[IBIS Ver]   3.2
[File name]   apollo7a.ibs
[File Rev]   0.2
[Date]   Wed Oct 23 16:15:15 CDT 2002
[Source]   File originated at Motorola Somerset Design Center.
|   Created by Jim Nissen.
[Notes]   This IBIS model is for the Apollo7 360CBGA ceramic package.
|   The driver and receiver models are characterized up to
|   2.5V mode on the data bus and 2.5V mode on the L3
|   interface. The convention is apollox.ibs, where x
|   is one of the configurations of data bus/L3 bus voltage
|   modes. Following is a table of the code for bus combinations:
|   IBIS model   Bus mode   L3 mode
|   apollo7a.ibs   2.5V   2.5V
|   apollo7b.ibs   2.5V   1.8V
|   apollo7c.ibs   2.5V   1.5V
|   apollo7d.ibs   1.8V   2.5V
|   apollo7e.ibs   1.8V   1.8V
|   apollo7f.ibs   1.8V   1.5V
|   apollo7g.ibs   1.5V   2.5V
|   apollo7h.ibs   1.5V   1.8V
|   apollo7i.ibs   1.5V   1.5V
[Disclaimer]   This information is for modeling purposes only and
|   is not guaranteed.
[Component]   Apollo7
[Manufacturer]  Motorola
[Package]
|   typ   min   max
R_pkg   0.0   0.0   0.0
L_pkg   0.0   0.0   0.0
C_pkg   0.0   0.0   0.0
[Pin]   signal_name   model_name   R_pin   L_pin   C_pin
A2   SRESET_B   busio   1E-016   1E-016   1E-016
A3   CKSTP_IN_B   busio   1E-016   1E-016   1E-016
A4   TDO   busio   1E-016   1E-016   1E-016
A5   TRST_B   rcvr   1E-016   1E-016   1E-016
A6   HPR_B   busio   1E-016   1E-016   1E-016
A7   PLL_CFG(4)   busio   1E-016   1E-016   1E-016
A9   PMON_OUT_B   busio   1E-016   1E-016   1E-016
A10   SYSCLK   busio   1E-016   1E-016   1E-016
A11   EXT_QUAL   busio   1E-016   1E-016   1E-016
A12   CHKS_B   busio   1E-016   1E-016   1E-016
A13   L3_DATA(59)   l3io   1E-016   1E-016   1E-016
A14   L3_DATA(61)   l3io   1E-016   1E-016   1E-016
A15   L3_DATA(56)   l3io   1E-016   1E-016   1E-016
A16   L3_DATA(36)   l3io   1E-016   1E-016   1E-016
A17   L3_DATA(50)   l3io   1E-016   1E-016   1E-016
A18   L3_DATA(58)   l3io   1E-016   1E-016   1E-016
A19   L3_DATA(38)   l3io   1E-016   1E-016   1E-016
B1   CKSTP_OUT_B   busio   1E-016   1E-016   1E-016
B2   HIT_B   busio   1E-016   1E-016   1E-016
B3   L2_TSTCLK   rcvr   1E-016   1E-016   1E-016
B6   IARTRY0_B   busio   1E-016   1E-016   1E-016
B7   BVSEL   rcvr   1E-016   1E-016   1E-016
B8   PLL_CFG(0)   busio   1E-016   1E-016   1E-016
B9   TDI   rcvr   1E-016   1E-016   1E-016
B10   SRW_B(0)   busio   1E-016   1E-016   1E-016
B11   A(35)   busio   1E-016   1E-016   1E-016
B12   A(32)   busio   1E-016   1E-016   1E-016
B13   L3_DATAP(6)   l3io   1E-016   1E-016   1E-016
B14   L3_DATAP(7)   l3io   1E-016   1E-016   1E-016
B15   L3_DATA(41)   l3io   1E-016   1E-016   1E-016
B16   L3_DATA(55)   l3io   1E-016   1E-016   1E-016
B17   L3_DATA(42)   l3io   1E-016   1E-016   1E-016
B18   L3_DATAP(4)   l3io   1E-016   1E-016   1E-016
B19   L3_DATA(37)   l3io   1E-016   1E-016   1E-016
C1   AP(0)   busio   1E-016   1E-016   1E-016
C4   A(33)   busio   1E-016   1E-016   1E-016
C5   TT(4)   busio   1E-016   1E-016   1E-016
C6   TCK   rcvr   1E-016   1E-016   1E-016
C7   PLL_CFG(2)   busio   1E-016   1E-016   1E-016
C8   PLL_CFG(1)   busio   1E-016   1E-016   1E-016
C9   MCP_B   busio   1E-016   1E-016   1E-016
C10   A(8)   busio   1E-016   1E-016   1E-016
C11   A(2)   busio   1E-016   1E-016   1E-016
C13   L3_DATA(63)   l3io   1E-016   1E-016   1E-016
C14   L3_DATA(57)   l3io   1E-016   1E-016   1E-016
C15   L3_DATA(49)   l3io   1E-016   1E-016   1E-016
C16   L3_DATA(44)   l3io   1E-016   1E-016   1E-016
C17   L3_DATA(43)   l3io   1E-016   1E-016   1E-016
C18   L3_DATA(35)   l3io   1E-016   1E-016   1E-016
C19   L3_DATA(32)   l3io   1E-016   1E-016   1E-016
D1   A(7)   busio   1E-016   1E-016   1E-016
D2   BR_B   busio   1E-016   1E-016   1E-016
D3   WT_B   busio   1E-016   1E-016   1E-016
D4   INT_B   busio   1E-016   1E-016   1E-016
D7   PLL_CFG(3)   busio   1E-016   1E-016   1E-016
D8   HRESET_B   busio   1E-016   1E-016   1E-016
D9   PMON_IN_B   busio   1E-016   1E-016   1E-016
D10   DX_B   busio   1E-016   1E-016   1E-016
D11   A(6)   busio   1E-016   1E-016   1E-016
D12   A(10)   busio   1E-016   1E-016   1E-016
D14   L3_DATA(39)   l3io   1E-016   1E-016   1E-016
D15   L3_DATA(33)   l3io   1E-016   1E-016   1E-016
D16   L3_ADDR(16)   l3io   1E-016   1E-016   1E-016
D17   L3_ADDR(15)   l3io   1E-016   1E-016   1E-016
D18   L3_ADDR(8)"   l3io   1E-016   1E-016   1E-016
D19   L3_ADDR(11)   l3io   1E-016   1E-016   1E-016
E1   TBEN   busio   1E-016   1E-016   1E-016
E2   GBL_B   busio   1E-016   1E-016   1E-016
E3   AP(1)   busio   1E-016   1E-016   1E-016
E4   SHD0_B   busio   1E-016   1E-016   1E-016
E5   TT(0)   busio   1E-016   1E-016   1E-016
E6   TT(1)   busio   1E-016   1E-016   1E-016
E7   TSIZ(2)   busio   1E-016   1E-016   1E-016
E8   LSSD_MODE_B   rcvr   1E-016   1E-016   1E-016
E9   TT(3)   busio   1E-016   1E-016   1E-016
E10   SRW_B(1)   busio   1E-016   1E-016   1E-016
E11   A(0)   busio   1E-016   1E-016   1E-016
E12   L3_DATAP(5)   l3io   1E-016   1E-016   1E-016
E13   L3_DATA(54)   l3io   1E-016   1E-016   1E-016
E14   L3_DATA(46)   l3io   1E-016   1E-016   1E-016
E15   L3_DATA(40)   l3io   1E-016   1E-016   1E-016
E16   L3_ADDR(14)   l3io   1E-016   1E-016   1E-016
E19   L3_ADDR(7)   l3io   1E-016   1E-016   1E-016
F1   TMS   rcvr   1E-016   1E-016   1E-016
F4   A(14)   busio   1E-016   1E-016   1E-016
F5   AP(3)   busio   1E-016   1E-016   1E-016
F6   TT(2)   busio   1E-016   1E-016   1E-016
F7   TSIZ(1)   busio   1E-016   1E-016   1E-016
F8   BMODE_B(1)   busio   1E-016   1E-016   1E-016
F9   SMI_B   busio   1E-016   1E-016   1E-016
F10   A(4)   busio   1E-016   1E-016   1E-016
F11   TBST_B   busio   1E-016   1E-016   1E-016
F12   L3_DATA(60)   l3io   1E-016   1E-016   1E-016
F13   L3_DATA(53)   l3io   1E-016   1E-016   1E-016
F14   L3_DATA(52)   l3io   1E-016   1E-016   1E-016
F15   L3_ADDR(12)   l3io   1E-016   1E-016   1E-016
F16   L3_ADDR(9)   l3io   1E-016   1E-016   1E-016
F17   L3_ADDR(1)   l3io   1E-016   1E-016   1E-016
F18   L3_ADDR(0)   l3io   1E-016   1E-016   1E-016
F19   L3_ADDR(2)   l3io   1E-016   1E-016   1E-016
G1   DTI(0)   busio   1E-016   1E-016   1E-016
G2   A(9)   busio   1E-016   1E-016   1E-016
G3   A(3)   busio   1E-016   1E-016   1E-016
G4   A(12)   busio   1E-016   1E-016   1E-016
G5   QACK_B   busio   1E-016   1E-016   1E-016
G6   TSIZ(0)   busio   1E-016   1E-016   1E-016
G7   AP(4)   busio   1E-016   1E-016   1E-016
G8   L1_TSTCLK   rcvr   1E-016   1E-016   1E-016
G9   BMODE_B(0)   busio   1E-016   1E-016   1E-016
G10   A(34)   busio   1E-016   1E-016   1E-016
G11   L3_DATA(62)   l3io   1E-016   1E-016   1E-016
G12   L3_DATA(51)   l3io   1E-016   1E-016   1E-016
G13   L3_DATA(45)   l3io   1E-016   1E-016   1E-016
G14   L3_DATA(48)   l3io   1E-016   1E-016   1E-016
G15   L3_DATA(34)   l3io   1E-016   1E-016   1E-016
G16   L3_ADDR(10)   l3io   1E-016   1E-016   1E-016
G19   L3_ADDR(13)   l3io   1E-016   1E-016   1E-016
H1   A(1)   busio   1E-016   1E-016   1E-016
H2   CLK_OUT   busio   1E-016   1E-016   1E-016
H5   SHD1_B   busio   1E-016   1E-016   1E-016
H6   AP(2)   busio   1E-016   1E-016   1E-016
H14   L3_DATA(47)   l3io   1E-016   1E-016   1E-016
H15   L3_DATA(23)   l3io   1E-016   1E-016   1E-016
H16   L3_ADDR(6)   l3io   1E-016   1E-016   1E-016
H17   L3_ADDR(5)   l3io   1E-016   1E-016   1E-016
H18   L3_ADDR(4)   l3io   1E-016   1E-016   1E-016
H19   L3_ADDR(3)   l3io   1E-016   1E-016   1E-016
J1   CI_B   busio   1E-016   1E-016   1E-016
J2   A(20)   busio   1E-016   1E-016   1E-016
J3   A(23)   busio   1E-016   1E-016   1E-016
J4   A(16)   busio   1E-016   1E-016   1E-016
J14   L3_DATA(17)   l3io   1E-016   1E-016   1E-016
J15   L3_DATA(20)   l3io   1E-016   1E-016   1E-016
J16   L3_DATA(22)   l3io   1E-016   1E-016   1E-016
J17   L3_DATA(30)   l3io   1E-016   1E-016   1E-016
J18   L3_DATA(18)   l3io   1E-016   1E-016   1E-016
J19   L3_DATA(19)   l3io   1E-016   1E-016   1E-016
K1   DTI(1)   busio   1E-016   1E-016   1E-016
K4   A(21)   busio   1E-016   1E-016   1E-016
K5   A(18)   busio   1E-016   1E-016   1E-016
K6   TA_B   busio   1E-016   1E-016   1E-016
K15   L3_DATA(16)   l3io   1E-016   1E-016   1E-016
K16   L3_DATA(31)   l3io   1E-016   1E-016   1E-016
K17   L3_DATAP(2)   l3io   1E-016   1E-016   1E-016
K18   L3_DATA(29)   l3io   1E-016   1E-016   1E-016
K19   L3_DATA(21)   l3io   1E-016   1E-016   1E-016
L1   TEA_B   busio   1E-016   1E-016   1E-016
L2   A(5)   busio   1E-016   1E-016   1E-016
L3   A(11)   busio   1E-016   1E-016   1E-016
L4   TS_B   busio   1E-016   1E-016   1E-016
L14   L3_DATA(15)   l3io   1E-016   1E-016   1E-016
L15   L3_DATA(1)   l3io   1E-016   1E-016   1E-016
L16   L3_DATA(24)   l3io   1E-016   1E-016   1E-016
L17   L3_DATA(14)   l3io   1E-016   1E-016   1E-016
L18   L3_DATA(28)   l3io   1E-016   1E-016   1E-016
L19   L3_DATA(27)   l3io   1E-016   1E-016   1E-016
M1   BG_B   busio   1E-016   1E-016   1E-016
M2   DBG_B   busio   1E-016   1E-016   1E-016
M5   A(24)   busio   1E-016   1E-016   1E-016
M6   DP(4)   busio   1E-016   1E-016   1E-016
M14   L3_DATA(5)   l3io   1E-016   1E-016   1E-016
M15   L3_DATA(13)   l3io   1E-016   1E-016   1E-016
M16   L3_DATA(10)   l3io   1E-016   1E-016   1E-016
M17   L3_DATA(6)   l3io   1E-016   1E-016   1E-016
M18   L3_DATA(26)   l3io   1E-016   1E-016   1E-016
M19   L3_DATA(9)   l3io   1E-016   1E-016   1E-016
N1   DTI(3)   busio   1E-016   1E-016   1E-016
N2   ARTRY_B   busio   1E-016   1E-016   1E-016
N3   A(26)   busio   1E-016   1E-016   1E-016
N4   A(22)   busio   1E-016   1E-016   1E-016
N5   A(30)   busio   1E-016   1E-016   1E-016
N8   DP(6)   busio   1E-016   1E-016   1E-016
N9   D(25)   busio   1E-016   1E-016   1E-016
N10   D(19)   busio   1E-016   1E-016   1E-016
N11   D(18)   busio   1E-016   1E-016   1E-016
N12   L3_DATAP(0)   l3io   1E-016   1E-016   1E-016
N13   L3_DATA(7)   l3io   1E-016   1E-016   1E-016
N14   L3_DATA(4)   l3io   1E-016   1E-016   1E-016
N15   L3_DATA(2)   l3io   1E-016   1E-016   1E-016
N16   L3_DATA(8)   l3io   1E-016   1E-016   1E-016
N17   L3_DATA(12)   l3io   1E-016   1E-016   1E-016
N18   L3_DATAP(1)   l3io   1E-016   1E-016   1E-016
N19   L3_DATAP(3)   l3io   1E-016   1E-016   1E-016
P1   DTI(2)   busio   1E-016   1E-016   1E-016
P4   QREQ_B   busio   1E-016   1E-016   1E-016
P5   A(25)   busio   1E-016   1E-016   1E-016
P6   D(60)   busio   1E-016   1E-016   1E-016
P7   D(38)   busio   1E-016   1E-016   1E-016
P10   D(26)   busio   1E-016   1E-016   1E-016
P13   D(11)   busio   1E-016   1E-016   1E-016
P14   D(7)   busio   1E-016   1E-016   1E-016
P15   L3_DATA(0)   l3io   1E-016   1E-016   1E-016
P16   L3_DATA(25)   l3io   1E-016   1E-016   1E-016
P17   D(40)   busio   1E-016   1E-016   1E-016
P18   L3_DATA(3)   l3io   1E-016   1E-016   1E-016
P19   L3_DATA(11)   l3io   1E-016   1E-016   1E-016
R1   AACK_B   busio   1E-016   1E-016   1E-016
R2   A(17)   busio   1E-016   1E-016   1E-016
R3   DRDY_B   busio   1E-016   1E-016   1E-016
R6   D(37)   busio   1E-016   1E-016   1E-016
R7   D(59)   busio   1E-016   1E-016   1E-016
R8   D(61)   busio   1E-016   1E-016   1E-016
R9   D(28)   busio   1E-016   1E-016   1E-016
R10   D(24)   busio   1E-016   1E-016   1E-016
R11   D(20)   busio   1E-016   1E-016   1E-016
R12   D(14)   busio   1E-016   1E-016   1E-016
R15   D(0)   busio   1E-016   1E-016   1E-016
R18   D(43)   busio   1E-016   1E-016   1E-016
R19   D(41)   busio   1E-016   1E-016   1E-016
T1   A(27)   busio   1E-016   1E-016   1E-016
T2   A(13)   busio   1E-016   1E-016   1E-016
T3   DP(0)   busio   1E-016   1E-016   1E-016
T4   DP(2)   busio   1E-016   1E-016   1E-016
T5   D(34)   busio   1E-016   1E-016   1E-016
T8   D(63)   busio   1E-016   1E-016   1E-016
T11   D(23)   busio   1E-016   1E-016   1E-016
T12   D(15)   busio   1E-016   1E-016   1E-016
T13   D(10)   busio   1E-016   1E-016   1E-016
T14   D(2)   busio   1E-016   1E-016   1E-016
T15   D(5)   busio   1E-016   1E-016   1E-016
T16   D(51)   busio   1E-016   1E-016   1E-016
T17   D(53)   busio   1E-016   1E-016   1E-016
T18   D(52)   busio   1E-016   1E-016   1E-016
T19   D(45)   busio   1E-016   1E-016   1E-016
U1   A(29)   busio   1E-016   1E-016   1E-016
U4   D(56)   busio   1E-016   1E-016   1E-016
U5   D(35)   busio   1E-016   1E-016   1E-016
U6   D(33)   busio   1E-016   1E-016   1E-016
U7   D(58)   busio   1E-016   1E-016   1E-016
U8   D(57)   busio   1E-016   1E-016   1E-016
U9   D(30)   busio   1E-016   1E-016   1E-016
U10   D(27)   busio   1E-016   1E-016   1E-016
U11   D(21)   busio   1E-016   1E-016   1E-016
U14   D(12)   busio   1E-016   1E-016   1E-016
U15   D(6)   busio   1E-016   1E-016   1E-016
U18   D(48)   busio   1E-016   1E-016   1E-016
U19   D(46)   busio   1E-016   1E-016   1E-016
V1   A(15)   busio   1E-016   1E-016   1E-016
V2   A(28)   busio   1E-016   1E-016   1E-016
V3   DP(5)   busio   1E-016   1E-016   1E-016
V6   D(39)   busio   1E-016   1E-016   1E-016
V9   D(31)   busio   1E-016   1E-016   1E-016
V12   D(17)   busio   1E-016   1E-016   1E-016
V13   D(8)   busio   1E-016   1E-016   1E-016
V16   D(3)   busio   1E-016   1E-016   1E-016
V17   D(55)   busio   1E-016   1E-016   1E-016
V18   D(42)   busio   1E-016   1E-016   1E-016
V19   D(44)   busio   1E-016   1E-016   1E-016
W1   A(31)   busio   1E-016   1E-016   1E-016
W2   A(19)   busio   1E-016   1E-016   1E-016
W3   D(54)   busio   1E-016   1E-016   1E-016
W4   DP(1)   busio   1E-016   1E-016   1E-016
W5   D(32)   busio   1E-016   1E-016   1E-016
W6   DP(7)   busio   1E-016   1E-016   1E-016
W7   D(36)   busio   1E-016   1E-016   1E-016
W8   D(62)   busio   1E-016   1E-016   1E-016
W9   DP(3)   busio   1E-016   1E-016   1E-016
W10   D(29)   busio   1E-016   1E-016   1E-016
W11   D(22)   busio   1E-016   1E-016   1E-016
W12   D(16)   busio   1E-016   1E-016   1E-016
W13   D(9)   busio   1E-016   1E-016   1E-016
W14   D(13)   busio   1E-016   1E-016   1E-016
W15   D(1)   busio   1E-016   1E-016   1E-016
W16   D(4)   busio   1E-016   1E-016   1E-016
W17   D(49)   busio   1E-016   1E-016   1E-016
W18   D(50)   busio   1E-016   1E-016   1E-016
W19   D(47)   busio   1E-016   1E-016   1E-016
|!!!![Package Model] 'name'  calls name
[Package Model] apollo7_360
[Define Package Model] apollo7_360
[Manufacturer] Motorola Inc.
[OEM] Motorola Inc.
[Description] Apollo7 360 CBGA Package T-Line pkg model
[Number Of Sections] 10
[Number Of Pins]  267
[Pin Numbers]
|Although any length unit can be used for Len, mm is used here.
|signal (1)SYSCLK
A10   Len=0 L=0.023752784n /
Len=0 L=0.0115888305n /
Len=10.910172 L=0.41228828n C=0.27619976p R=0.045776114 /
Len=0 L=0.0115888305n /
Len=0 L=0.0115888305n /
Len=0 L=0.0115888305n /
Len=0 L=0.0115888305n /
Len=0 L=0.027n /
|signal (2)EXT_QUAL
A11   Len=0 L=0.023752784n /
Len=0 L=0.0115888305n /
Len=10.207413 L=0.41011378n C=0.27773488p R=0.04516712 /
Len=0 L=0.0115888305n /
Len=0 L=0.0115888305n /
Len=0 L=0.0115888305n /
Len=0 L=0.0115888305n /
Len=0 L=0.027n /
|signal (3)CHKS_B
A12   Len=0 L=0.023752784n /
Len=0 L=0.0115888305n /
Len=0 L=0.0115888305n /
Len=0 L=0.0115888305n /
Len=12.901163 L=0.4005851n C=0.2846683p R=0.04260898 /
Len=0 L=0.0115888305n /
Len=0 L=0.0115888305n /
Len=0 L=0.027n /
|signal (4)L3_DATA(59)
A13   Len=0 L=0.023752784n /
Len=0 L=0.0115888305n /
Len=0 L=0.0115888305n /
Len=0 L=0.0115888305n /
Len=5.8014994 L=0.42097718n C=0.2702314p R=0.04830918 /
Len=0 L=0.0115888305n /
Len=0 L=0.0115888305n /
Len=5.8287997 L=0.4658248n C=0.12673753p R=0.041152265 /
Len=0 L=0.027n /
|signal (5)L3_DATA(61)
A14   Len=0 L=0.023752784n /
Len=0 L=0.0115888305n /
Len=11.64697 L=0.40967372n C=0.27804765p R=0.045045044 /
Len=0 L=0.0115888305n /
Len=0 L=0.0115888305n /
Len=0 L=0.0115888305n /
Len=0 L=0.0115888305n /
Len=0 L=0.027n /
|signal (6)L3_DATA(56)
A15   Len=0 L=0.023752784n /
Len=0 L=0.0115888305n /
Len=0 L=0.0115888305n /
Len=0 L=0.0115888305n /
Len=0 L=0.0115888305n /
Len=0 L=0.0115888305n /
Len=14.642346 L=0.4886838n C=0.120809175p R=0.047340576 /
Len=0 L=0.027n /
|signal (7)L3_DATA(36)
A16   Len=0 L=0.023752784n /
Len=0 L=0.0115888305n /
Len=0 L=0.0115888305n /
Len=0 L=0.0115888305n /
Len=9.291906 L=0.41293234n C=0.27574828p R=0.045958366 /
Len=0 L=0.0115888305n /
Len=0 L=0.0115888305n /
Len=5.9719596 L=0.4658248n C=0.12673753p R=0.041152265 /
Len=0 L=0.027n /
|signal (8)L3_DATA(50)
A17   Len=0 L=0.023752784n /
Len=0 L=0.0115888305n /
Len=0 L=0.0115888305n /
Len=0 L=0.0115888305n /
Len=0 L=0.0115888305n /
Len=0 L=0.0115888305n /
Len=17.10347 L=0.4950636n C=0.119252324p R=0.049261082 /
Len=0 L=0.027n /
|signal (9)L3_DATA(58)
A18   Len=0 L=0.023752784n /
Len=0 L=0.0115888305n /
Len=0 L=0.0115888305n /
Len=0 L=0.0115888305n /
Len=0 L=0.0115888305n /
Len=0 L=0.0115888305n /
Len=18.881626 L=0.4838978n C=0.12200403p R=0.045958366 /
Len=0 L=0.027n /
|signal (10)L3_DATA(38)
A19   Len=0 L=0.023752784n /
Len=0 L=0.0115888305n /
Len=15.105156 L=0.409125n C=0.2784386p R=0.044893377 /
Len=0 L=0.0115888305n /
Len=0 L=0.0115888305n /
Len=0 L=0.0115888305n /
Len=0 L=0.0115888305n /
Len=0 L=0.027n /
|signal (11)SRESET_B
A2   Len=0 L=0.023752784n /
Len=0 L=0.0115888305n /
Len=11.204234 L=0.409125n C=0.2784386p R=0.044893377 /
Len=0 L=0.0115888305n /
Len=0 L=0.0115888305n /
Len=0 L=0.0115888305n /
Len=0 L=0.0115888305n /
Len=0 L=0.027n /
|signal (12)CKSTP_IN_B
A3   Len=0 L=0.023752784n /
Len=0 L=0.0115888305n /
Len=8.04229 L=0.44115186n C=0.25732118p R=0.054869685 /
Len=0 L=0.0115888305n /
Len=0 L=0.0115888305n /
Len=3.6205425 L=0.3948527n C=0.28900883p R=0.041152265 /
Len=0 L=0.0115888305n /
Len=0 L=0.0115888305n /
Len=0 L=0.027n /
|signal (13)TDO
A4   Len=0 L=0.023752784n /
Len=0 L=0.0115888305n /
Len=0 L=0.0115888305n /
Len=0 L=0.0115888305n /
Len=2.6897635 L=0.4182054n C=0.27210706p R=0.04748338 /
Len=0 L=0.0115888305n /
Len=0 L=0.0115888305n /
Len=15.088556 L=0.4658248n C=0.12673753p R=0.041152265 /
Len=0 L=0.027n /
|signal (14)TRST_B
A5   Len=0 L=0.023752784n /
Len=0 L=0.0115888305n /
Len=11.024857 L=0.3948527n C=0.28900883p R=0.041152265 /
Len=0 L=0.0115888305n /
Len=0 L=0.0115888305n /
Len=0 L=0.0115888305n /
Len=0 L=0.0115888305n /
Len=0 L=0.027n /
|signal (15)HPR_B
A6   Len=0 L=0.023752784n /
Len=0 L=0.0115888305n /
Len=8.710801 L=0.41188377n C=0.276484p R=0.045662098 /
Len=0 L=0.0115888305n /
Len=0 L=0.0115888305n /
Len=0 L=0.0115888305n /
Len=0 L=0.0115888305n /
Len=0 L=0.027n /
|signal (16)PLL_CFG(4)
A7   Len=0 L=0.023752784n /
Len=0 L=0.0115888305n /
Len=10.387514 L=0.41666302n C=0.27316216p R=0.047031157 /
Len=0 L=0.0115888305n /
Len=0 L=0.0115888305n /
Len=0 L=0.0115888305n /
Len=0 L=0.0115888305n /
Len=0 L=0.027n /
|signal (17)PMON_OUT_B
A9   Len=0 L=0.023752784n /
Len=0 L=0.0115888305n /
Len=9.733491 L=0.41884163n C=0.27167422p R=0.047671434 /
Len=0 L=0.0115888305n /
Len=0 L=0.0115888305n /
Len=4.389836 L=0.3948527n C=0.28900883p R=0.041152265 /
Len=0 L=0.0115888305n /
Len=0 L=0.0115888305n /
Len=0 L=0.027n /
|signal (18)CKSTP_OUT_B
B1   Len=0 L=0.023752784n /
Len=0 L=0.0115888305n /
Len=0 L=0.0115888305n /
Len=0 L=0.0115888305n /
Len=11.503042 L=0.3948527n C=0.28900883p R=0.041152265 /
Len=0 L=0.0115888305n /
Len=0 L=0.0115888305n /
Len=0 L=0.027n /
|signal (19)SRW_B(0)
B10   Len=0 L=0.023752784n /
Len=0 L=0.0115888305n /
Len=0 L=0.0115888305n /
Len=0 L=0.0115888305n /
Len=2.2702632 L=0.43544444n C=0.26084659p R=0.052910052 /
Len=0 L=0.0115888305n /
Len=0 L=0.0115888305n /
Len=7.4049344 L=0.46994686n C=0.12562588p R=0.04219409 /
Len=0 L=0.027n /
|signal (20)A(35)
B11   Len=0 L=0.023752784n /
Len=0 L=0.0115888305n /
Len=0 L=0.0115888305n /
Len=0 L=0.0115888305n /
Len=3.4159508 L=0.44380108n C=0.25571698p R=0.05580923 /
Len=0 L=0.0115888305n /
Len=0 L=0.0115888305n /
Len=10.56159 L=0.49349537n C=0.11963128p R=0.048780486 /
Len=0 L=0.027n /
|signal (21)A(32)
B12   Len=0 L=0.023752784n /
Len=0 L=0.0115888305n /
Len=0 L=0.0115888305n /
Len=0 L=0.0115888305n /
Len=13.818225 L=0.4141186n C=0.27492067p R=0.046296295 /
Len=0 L=0.0115888305n /
Len=0 L=0.0115888305n /
Len=0 L=0.027n /
|signal (22)L3_DATAP(6)
B13   Len=0 L=0.023752784n /
Len=0 L=0.0115888305n /
Len=9.38731 L=0.40748784n C=0.27961165p R=0.04444444 /
Len=0 L=0.0115888305n /
Len=0 L=0.0115888305n /
Len=0 L=0.0115888305n /
Len=0 L=0.0115888305n /
Len=0 L=0.027n /
|signal (23)L3_DATAP(7)
B14   Len=0 L=0.023752784n /
Len=0 L=0.0115888305n /
Len=10.790969 L=0.40233743n C=0.28336737p R=0.043066323 /
Len=0 L=0.0115888305n /
Len=0 L=0.0115888305n /
Len=0 L=0.0115888305n /
Len=0 L=0.0115888305n /
Len=0 L=0.027n /
|signal (24)L3_DATA(41)
B15   Len=0 L=0.023752784n /
Len=0 L=0.0115888305n /
Len=0 L=0.0115888305n /
Len=0 L=0.0115888305n /
Len=6.8211646 L=0.43544444n C=0.26084659p R=0.052910052 /
Len=0 L=0.0115888305n /
Len=0 L=0.0115888305n /
Len=12.433501 L=0.4733069n C=0.12473405p R=0.043066323 /
Len=0 L=0.027n /
|signal (25)L3_DATA(55)
B16   Len=0 L=0.023752784n /
Len=0 L=0.0115888305n /
Len=0 L=0.0115888305n /
Len=0 L=0.0115888305n /
Len=9.6519165 L=0.4042533n C=0.28195858p R=0.043572985 /
Len=0 L=0.0115888305n /
Len=0 L=0.0115888305n /
Len=4.6283216 L=0.4658248n C=0.12673753p R=0.041152265 /
Len=0 L=0.027n /
|signal (26)L3_DATA(42)
B17   Len=0 L=0.023752784n /
Len=0 L=0.0115888305n /
Len=9.0457535 L=0.42378795n C=0.26835555p R=0.049164206 /
Len=0 L=0.0115888305n /
Len=0 L=0.0115888305n /
Len=1.4367893 L=0.3948527n C=0.28900883p R=0.041152265 /
Len=0 L=0.0115888305n /
Len=0 L=0.0115888305n /
Len=4.5466576 L=0.4658248n C=0.12673753p R=0.041152265 /
Len=0 L=0.027n /
|signal (27)L3_DATAP(4)
B18   Len=0 L=0.023752784n /
Len=0 L=0.0115888305n /
Len=0 L=0.0115888305n /
Len=0 L=0.0115888305n /
Len=10.123784 L=0.42807978n C=0.26554102p R=0.05050505 /
Len=0 L=0.0115888305n /
Len=0 L=0.0115888305n /
Len=10.859214 L=0.4658248n C=0.12673753p R=0.041152265 /
Len=0 L=0.027n /
|signal (28)L3_DATA(37)
B19   Len=0 L=0.023752784n /
Len=0 L=0.0115888305n /
Len=14.317915 L=0.40563312n C=0.2809526p R=0.043942247 /
Len=0 L=0.0115888305n /
Len=0 L=0.0115888305n /
Len=0 L=0.0115888305n /
Len=0 L=0.0115888305n /
Len=0 L=0.027n /
|signal (29)HIT_B
B2   Len=0 L=0.023752784n /
Len=0 L=0.0115888305n /
Len=10.97225 L=0.4107757n C=0.2772658p R=0.045351475 /
Len=0 L=0.0115888305n /
Len=0 L=0.0115888305n /
Len=0 L=0.0115888305n /
Len=0 L=0.0115888305n /
Len=0 L=0.027n /
|signal (30)L2_TSTCLK
B3   Len=0 L=0.023752784n /
Len=0 L=0.0115888305n /
Len=11.309037 L=0.40233743n C=0.28336737p R=0.043066323 /
Len=0 L=0.0115888305n /
Len=0 L=0.0115888305n /
Len=2.095935 L=0.3948527n C=0.28900883p R=0.041152265 /
Len=0 L=0.0115888305n /
Len=0 L=0.0115888305n /
Len=0 L=0.027n /
|signal (31)IARTRY0_B
B6   Len=0 L=0.023752784n /
Len=0 L=0.0115888305n /
Len=7.5469265 L=0.40748784n C=0.27961165p R=0.04444444 /
Len=0 L=0.0115888305n /
Len=0 L=0.0115888305n /
Len=4.81949 L=0.3948527n C=0.28900883p R=0.041152265 /
Len=0 L=0.0115888305n /
Len=0 L=0.0115888305n /
Len=0 L=0.027n /
|signal (32)BVSEL
B7   Len=0 L=0.023752784n /
Len=0 L=0.0115888305n /
Len=6.138204 L=0.4141186n C=0.27492067p R=0.046296295 /
Len=0 L=0.0115888305n /
Len=0 L=0.0115888305n /
Len=2.185389 L=0.3948527n C=0.28900883p R=0.041152265 /
Len=0 L=0.0115888305n /
Len=0 L=0.0115888305n /
Len=0 L=0.027n /
|signal (33)PLL_CFG(0)
B8   Len=0 L=0.023752784n /
Len=0 L=0.0115888305n /
Len=6.500624 L=0.42097718n C=0.2702314p R=0.04830918 /
Len=0 L=0.0115888305n /
Len=0 L=0.0115888305n /
Len=0 L=0.0115888305n /
Len=0 L=0.0115888305n /
Len=0 L=0.027n /
|signal (34)TDI
B9   Len=0 L=0.023752784n /
Len=0 L=0.0115888305n /
Len=7.5004077 L=0.41228828n C=0.27619976p R=0.045776114 /
Len=0 L=0.0115888305n /
Len=0 L=0.0115888305n /
Len=0 L=0.0115888305n /
Len=0 L=0.0115888305n /
Len=0 L=0.027n /
|signal (35)AP(0)
C1   Len=0 L=0.023752784n /
Len=0 L=0.0115888305n /
Len=0 L=0.0115888305n /
Len=0 L=0.0115888305n /
Len=13.965541 L=0.42171302n C=0.26973775p R=0.04853129 /
Len=0 L=0.0115888305n /
Len=0 L=0.0115888305n /
Len=0 L=0.027n /
|signal (36)A(8)
C10   Len=0 L=0.023752784n /
Len=0 L=0.0115888305n /
Len=0 L=0.0115888305n /
Len=0 L=0.0115888305n /
Len=3.6626647 L=0.43544444n C=0.26084659p R=0.052910052 /
Len=0 L=0.0115888305n /
Len=0 L=0.0115888305n /
Len=7.3477516 L=0.4912431n C=0.12017977p R=0.048100047 /
Len=0 L=0.027n /
|signal (37)A(2)
C11   Len=0 L=0.023752784n /
Len=0 L=0.0115888305n /
Len=7.434594 L=0.42378795n C=0.26835555p R=0.049164206 /
Len=0 L=0.0115888305n /
Len=0 L=0.0115888305n /
Len=6.439806 L=0.3948527n C=0.28900883p R=0.041152265 /
Len=0 L=0.0115888305n /
Len=0 L=0.0115888305n /
Len=0 L=0.027n /
|signal (38)L3_DATA(63)
C13   Len=0 L=0.023752784n /
Len=0 L=0.0115888305n /
Len=0 L=0.0115888305n /
Len=0 L=0.0115888305n /
Len=7.2843323 L=0.41971248n C=0.27108398p R=0.04793028 /
Len=0 L=0.0115888305n /
Len=0 L=0.0115888305n /
Len=2.9857688 L=0.4658248n C=0.12673753p R=0.041152265 /
Len=0 L=0.027n /
|signal (39)L3_DATA(57)
C14   Len=0 L=0.023752784n /
Len=0 L=0.0115888305n /
Len=0 L=0.0115888305n /
Len=0 L=0.0115888305n /
Len=0 L=0.0115888305n /
Len=0 L=0.0115888305n /
Len=9.871671 L=0.50107294n C=0.11782214p R=0.051156126 /
Len=0 L=0.027n /
|signal (40)L3_DATA(49)
C15   Len=0 L=0.023752784n /
Len=0 L=0.0115888305n /
Len=5.5947742 L=0.43544444n C=0.26084659p R=0.052910052 /
Len=0 L=0.0115888305n /
Len=0 L=0.0115888305n /
Len=0 L=0.0115888305n /
Len=0 L=0.0115888305n /
Len=10.48825 L=0.47170827n C=0.12515678p R=0.04264871 /
Len=0 L=0.027n /
|signal (41)L3_DATA(44)
C16   Len=0 L=0.023752784n /
Len=0 L=0.0115888305n /
Len=0 L=0.0115888305n /
Len=0 L=0.0115888305n /
Len=7.796008 L=0.4095047n C=0.27816793p R=0.04499827 /
Len=0 L=0.0115888305n /
Len=0 L=0.0115888305n /
Len=4.4824214 L=0.4658248n C=0.12673753p R=0.041152265 /
Len=0 L=0.027n /
|signal (42)L3_DATA(43)
C17   Len=0 L=0.023752784n /
Len=0 L=0.0115888305n /
Len=0 L=0.0115888305n /
Len=0 L=0.0115888305n /
Len=12.921658 L=0.41305688n C=0.27566117p R=0.045993708 /
Len=0 L=0.0115888305n /
Len=0 L=0.0115888305n /
Len=0 L=0.027n /
|signal (43)L3_DATA(35)
C18   Len=0 L=0.023752784n /
Len=0 L=0.0115888305n /
Len=11.989653 L=0.40563312n C=0.2809526p R=0.043942247 /
Len=0 L=0.0115888305n /
Len=0 L=0.0115888305n /
Len=0 L=0.0115888305n /
Len=0 L=0.0115888305n /
Len=0 L=0.027n /
|signal (44)L3_DATA(32)
C19   Len=0 L=0.023752784n /
Len=0 L=0.0115888305n /
Len=6.932434 L=0.43076158n C=0.26381212p R=0.051365234 /
Len=0 L=0.0115888305n /
Len=0 L=0.0115888305n /
Len=5.879125 L=0.3948527n C=0.28900883p R=0.041152265 /
Len=0 L=0.0115888305n /
Len=0 L=0.0115888305n /
Len=10.283896 L=0.4658248n C=0.12673753p R=0.041152265 /
Len=0 L=0.027n /
|signal (45)A(33)
C4   Len=0 L=0.023752784n /
Len=0 L=0.0115888305n /
Len=0 L=0.0115888305n /
Len=0 L=0.0115888305n /
Len=5.6502595 L=0.40748784n C=0.27961165p R=0.04444444 /
Len=0 L=0.0115888305n /
Len=0 L=0.0115888305n /
Len=4.33065 L=0.4658248n C=0.12673753p R=0.041152265 /
Len=0 L=0.027n /
|signal (46)TT(4)
C5   Len=0 L=0.023752784n /
Len=0 L=0.0115888305n /
Len=0.96351683 L=0.44309118n C=0.25614488p R=0.055555556 /
Len=0 L=0.0115888305n /
Len=0 L=0.0115888305n /
Len=0 L=0.0115888305n /
Len=0 L=0.0115888305n /
Len=7.7490196 L=0.4658248n C=0.12673753p R=0.041152265 /
Len=0 L=0.027n /
|signal (47)TCK
C6   Len=0 L=0.023752784n /
Len=0 L=0.0115888305n /
Len=7.927365 L=0.4333124n C=0.26218843p R=0.05219985 /
Len=0 L=0.0115888305n /
Len=0 L=0.0115888305n /
Len=0 L=0.0115888305n /
Len=0 L=0.0115888305n /
Len=0 L=0.027n /
|signal (48)PLL_CFG(2)
C7   Len=0 L=0.023752784n /
Len=0 L=0.0115888305n /
Len=5.729875 L=0.41228828n C=0.27619976p R=0.045776114 /
Len=0 L=0.0115888305n /
Len=0 L=0.0115888305n /
Len=0 L=0.0115888305n /
Len=0 L=0.0115888305n /
Len=0 L=0.027n /
|signal (49)PLL_CFG(1)
C8   Len=0 L=0.023752784n /
Len=0 L=0.0115888305n /
Len=5.4456906 L=0.4313937n C=0.2634079p R=0.051570557 /
Len=0 L=0.0115888305n /
Len=0 L=0.0115888305n /
Len=0 L=0.0115888305n /
Len=0 L=0.0115888305n /
Len=0 L=0.027n /
|signal (50)MCP_B
C9   Len=0 L=0.023752784n /
Len=0 L=0.0115888305n /
Len=0 L=0.0115888305n /
Len=0 L=0.0115888305n /
Len=0 L=0.0115888305n /
Len=0 L=0.0115888305n /
Len=8.329084 L=0.48221594n C=0.12242956p R=0.04548408 /
Len=0 L=0.027n /
|signal (51)A(7)
D1   Len=0 L=0.023752784n /
Len=0 L=0.0115888305n /
Len=11.060167 L=0.42205358n C=0.26950994p R=0.04863449 /
Len=0 L=0.0115888305n /
Len=0 L=0.0115888305n /
Len=0 L=0.0115888305n /
Len=0 L=0.0115888305n /
Len=0 L=0.027n /
|signal (52)DX_B
D10   Len=0 L=0.023752784n /
Len=0 L=0.0115888305n /
Len=5.415398 L=0.42602456n C=0.2668814p R=0.04985755 /
Len=0 L=0.0115888305n /
Len=0 L=0.0115888305n /
Len=0 L=0.0115888305n /
Len=0 L=0.0115888305n /
Len=0 L=0.027n /
|signal (53)A(6)
D11   Len=0 L=0.023752784n /
Len=0 L=0.0115888305n /
Len=0 L=0.0115888305n /
Len=0 L=0.0115888305n /
Len=4.097878 L=0.43544444n C=0.26084659p R=0.052910052 /
Len=0 L=0.0115888305n /
Len=0 L=0.0115888305n /
Len=7.3189435 L=0.49193937n C=0.120009676p R=0.04830918 /
Len=0 L=0.027n /
|signal (54)A(10)
D12   Len=0 L=0.023752784n /
Len=0 L=0.0115888305n /
Len=0 L=0.0115888305n /
Len=0 L=0.0115888305n /
Len=3.7324407 L=0.43544444n C=0.26084659p R=0.052910052 /
Len=0 L=0.0115888305n /
Len=0 L=0.0115888305n /
Len=7.3175383 L=0.48664492n C=0.12131532p R=0.046745777 /
Len=0 L=0.027n /
|signal (55)L3_DATA(39)
D14   Len=0 L=0.023752784n /
Len=0 L=0.0115888305n /
Len=4.221292 L=0.43544444n C=0.26084659p R=0.052910052 /
Len=0 L=0.0115888305n /
Len=0 L=0.0115888305n /
Len=0 L=0.0115888305n /
Len=0 L=0.0115888305n /
Len=8.922007 L=0.48508358n C=0.1217058p R=0.046296295 /
Len=0 L=0.027n /
|signal (56)L3_DATA(33)
D15   Len=0 L=0.023752784n /
Len=0 L=0.0115888305n /
Len=7.8460646 L=0.41124985n C=0.27693075p R=0.04548408 /
Len=0 L=0.0115888305n /
Len=0 L=0.0115888305n /
Len=0 L=0.0115888305n /
Len=0 L=0.0115888305n /
Len=0 L=0.027n /
|signal (57)L3_ADDR(16)
D16   Len=0 L=0.023752784n /
Len=0 L=0.0115888305n /
Len=7.8873067 L=0.41124985n C=0.27693075p R=0.04548408 /
Len=0 L=0.0115888305n /
Len=0 L=0.0115888305n /
Len=0 L=0.0115888305n /
Len=0 L=0.0115888305n /
Len=0 L=0.027n /
|signal (58)L3_ADDR(15)
D17   Len=0 L=0.023752784n /
Len=0 L=0.0115888305n /
Len=9.894904 L=0.40233743n C=0.28336737p R=0.043066323 /
Len=0 L=0.0115888305n /
Len=0 L=0.0115888305n /
Len=0 L=0.0115888305n /
Len=0 L=0.0115888305n /
Len=0 L=0.027n /
|signal (59)L3_ADDR(8)
D18   Len=0 L=0.023752784n /
Len=0 L=0.0115888305n /
Len=9.783769 L=0.4095047n C=0.27816793p R=0.04499827 /
Len=0 L=0.0115888305n /
Len=0 L=0.0115888305n /
Len=0 L=0.0115888305n /
Len=0 L=0.0115888305n /
Len=0 L=0.027n /
|signal (60)L3_ADDR(11)
D19   Len=0 L=0.023752784n /
Len=0 L=0.0115888305n /
Len=9.826237 L=0.4086772n C=0.2787585p R=0.044770043 /
Len=0 L=0.0115888305n /
Len=0 L=0.0115888305n /
Len=1.3420033 L=0.3948527n C=0.28900883p R=0.041152265 /
Len=0 L=0.0115888305n /
Len=0 L=0.0115888305n /
Len=0 L=0.027n /
|signal (61)BR_B
D2   Len=0 L=0.023752784n /
Len=0 L=0.0115888305n /
Len=6.2067943 L=0.425318n C=0.2673453p R=0.049637266 /
Len=0 L=0.0115888305n /
Len=0 L=0.0115888305n /
Len=4.9862037 L=0.3948527n C=0.28900883p R=0.041152265 /
Len=0 L=0.0115888305n /
Len=0 L=0.0115888305n /
Len=0 L=0.027n /
|signal (62)WT_B
D3   Len=0 L=0.023752784n /
Len=0 L=0.0115888305n /
Len=2.5558584 L=0.40563312n C=0.2809526p R=0.043942247 /
Len=0 L=0.0115888305n /
Len=0 L=0.0115888305n /
Len=0 L=0.0115888305n /
Len=0 L=0.0115888305n /
Len=11.97358 L=0.4658248n C=0.12673753p R=0.041152265 /
Len=0 L=0.027n /
|signal (63)INT_B
D4   Len=0 L=0.023752784n /
Len=0 L=0.0115888305n /
Len=0 L=0.0115888305n /
Len=0 L=0.0115888305n /
Len=1.7920032 L=0.4309931n C=0.2636639p R=0.05144033 /
Len=0 L=0.0115888305n /
Len=0 L=0.0115888305n /
Len=10.752604 L=0.4658248n C=0.12673753p R=0.041152265 /
Len=0 L=0.027n /
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[End Package Model]
| Models and submodels in the file (3): busio (I/O), rcvr (Input), l3io (I/O)
